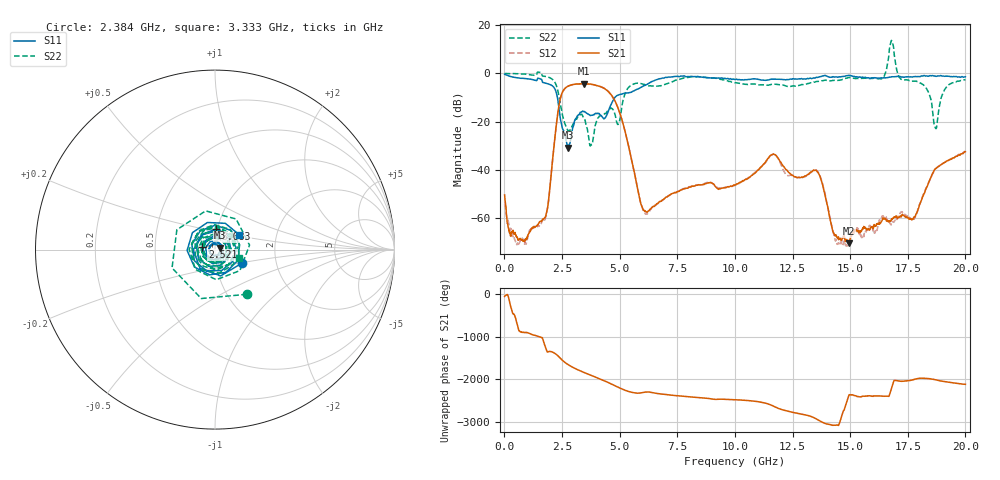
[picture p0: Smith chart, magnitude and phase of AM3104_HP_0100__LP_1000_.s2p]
!Created with skrf (http://scikit-rf.org).
# Hz S RI R 50.0
!freq ReS11 ImS11 ReS21 ImS21 ReS12 ImS12 ReS22 ImS22
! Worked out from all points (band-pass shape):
!   1601 points, 10 MHz to 20 GHz, reference 50 ohm
!   highest |S21| = -4.27 dB at 3.433 GHz (marker M1); lowest = -70.3 dB at 14.95 GHz (marker M2)
!   |S21| within 3 dB of the highest: 2.545 GHz to 4.487 GHz (1.942 GHz wide, 55.2 % of centre)
!   lowest |S11| = -30.8 dB at 2.771 GHz (marker M3), VSWR 1.06, Z = 52.7 + j1.15 ohm
!   |S11| at or under -10 dB: 2.301 GHz to 4.789 GHz (2.488 GHz wide, 70.2 % of centre)
!   |S22| runs from -30.0 to 13.7 dB; largest |S21 - S12| = 0.044
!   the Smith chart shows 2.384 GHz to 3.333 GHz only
!   S11 on the Smith chart (normalised r, x): 2.384 GHz: 1.33, -0.21; 2.521 GHz: 0.87, +0.03; 3.083 GHz: 0.99, +0.23; 3.333 GHz: 1.29, +0.22
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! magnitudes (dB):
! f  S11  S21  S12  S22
! 10 MHz  -0.4  -50.3  -54.2  0.0
! 672.2 MHz  -2.0  -68.5  -69.8  -0.2
! 1.722 GHz  -3.8  -60.1  -60.3  -1.1
! 2.384 GHz  -15.5  -12.4  -12.5  -10.3
! 2.521 GHz  -22.9  -7.7  -7.7  -17.3
! 2.771 GHz  -30.8  -5.2  -5.3  -23.8
! 3.083 GHz  -18.9  -4.4  -4.4  -19.1
! 3.333 GHz  -16.0  -4.3  -4.4  -17.0
! 3.346 GHz  -15.9  -4.3  -4.4  -16.9
! 3.433 GHz  -15.8  -4.3  -4.3  -18.4
! 3.758 GHz  -17.4  -4.5  -4.5  -29.4
! 4.708 GHz  -11.3  -9.8  -10.0  -14.9
! 6.019 GHz  -5.2  -56.4  -56.6  -4.5
! 6.682 GHz  -2.3  -53.5  -53.6  -5.3
! 10.01 GHz  -2.5  -46.3  -46.4  -3.9
! 11.64 GHz  -2.4  -33.6  -33.5  -4.4
! 13.34 GHz  -2.1  -40.6  -40.6  -3.9
! 14.95 GHz  -0.8  -70.3  -70.3  -1.7
! 16.68 GHz  -1.6  -61.3  -61.2  7.3
! 17.79 GHz  -1.3  -59.4  -60.1  -3.1
! 18.7 GHz  -1.2  -39.4  -39.5  -22.6
! 20 GHz  -1.4  -32.4  -32.2  -2.6
